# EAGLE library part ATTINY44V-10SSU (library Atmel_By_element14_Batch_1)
8-bit Microcontroller with Bytes In-System Programmable Flash
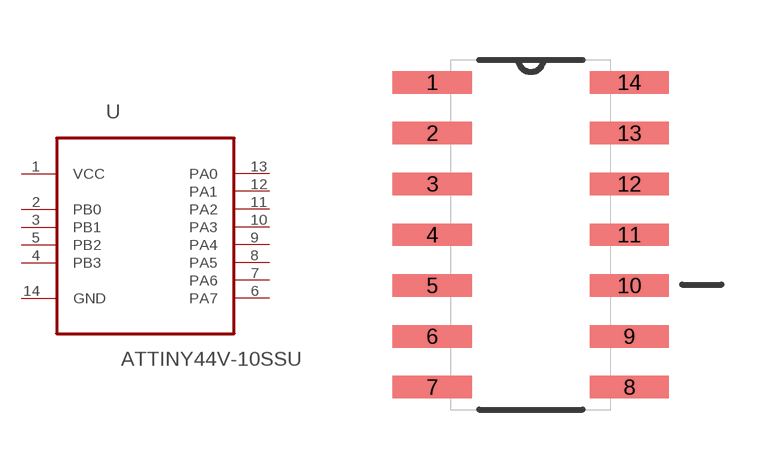
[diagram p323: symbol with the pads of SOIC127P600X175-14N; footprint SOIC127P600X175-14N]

Designator prefix U

## ATTINY44V-10SSU (MPN: ATTINY44V-10SSU; OC_FARNELL: 1455154; OC_NEWARK: 58M3789; PACKAGE: SOIC-14; SUPPLIER: Atmel)  [SOIC127P600X175-14N]
1  VCC  pwr
2  PB0
3  PB1
4  PB3
5  PB2
6  PA7
7  PA6
8  PA5
9  PA4
10  PA3
11  PA2
12  PA1
13  PA0
14  GND  pas

## Footprint SOIC127P600X175-14N (pad centres in mm)
smd 1.981 x 0.559: 1 -2.464,3.81; 2 -2.464,2.54; 3 -2.464,1.27; 4 -2.464,0; 5 -2.464,-1.27; 6 -2.464,-2.54; 7 -2.464,-3.81; 8 2.464,-3.81; 9 2.464,-2.54; 10 2.464,-1.27; 11 2.464,0; 12 2.464,1.27; 13 2.464,2.54; 14 2.464,3.81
